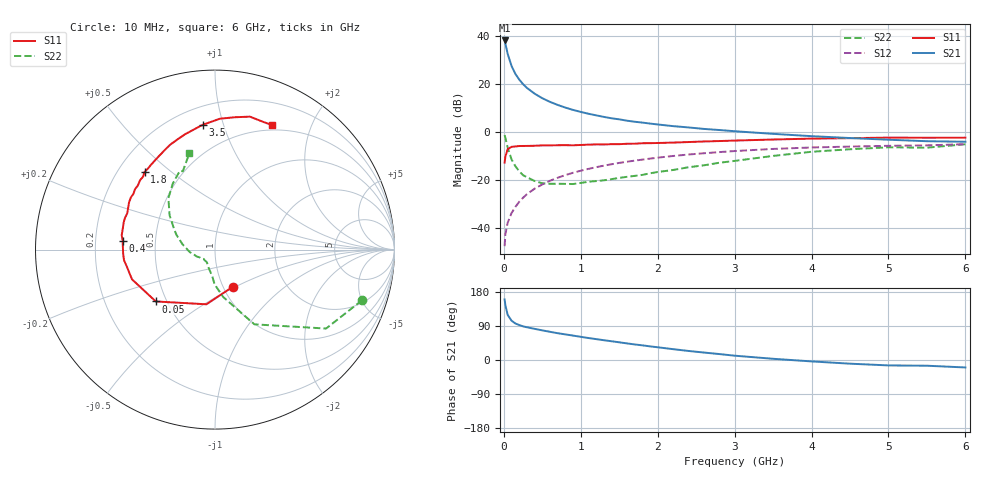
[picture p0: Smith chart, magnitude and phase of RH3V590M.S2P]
! SIEMENS Small Signal Semiconductors
! BFR106
! Si NPN RF Bipolar Junction Transistor in SOT23
! VCE = 3.5 V  IC = 90 mA
! Common Emitter S-Parameters:  August  1996
# GHz  S  MA  R  50
!  f  S11  S21  S12  S22
! GHz  MAG  ANG  MAG  ANG  MAG  ANG  MAG  ANG
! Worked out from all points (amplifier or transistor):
!   36 points, 10 MHz to 6 GHz, reference 50 ohm
!   highest |S21| = 38.3 dB at 10 MHz (marker M1)
!   |S21| within 3 dB of that: start of sweep to 31.7 MHz
!   unconditionally stable (mu >= 1): 167.4 MHz to 2.468 GHz; 5.445 GHz to end of sweep
!   at 250 MHz: K = 1.06, MAG = 22.3 dB, |S12| = -27.5 dB
!   at 1.4 GHz: K = 1.06, MAG = 8.1 dB, |S12| = -13.5 dB
!   at 6 GHz: K = 1.00, MAG = 0.3 dB, |S12| = -5.1 dB
!   S11 on the Smith chart (normalised r, x): 10 MHz: 1.11, -0.48; 50 MHz: 0.44, -0.31; 400 MHz: 0.32, +0.04; 1.8 GHz: 0.31, +0.41; 3.5 GHz: 0.31, +0.85; 6 GHz: 0.44, +1.47
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0.01  0.2292 -64.2  82.62 159.9  0.0041 78.1  0.8664 -19.0
0.02  0.3084 -98.9  70.99 144.5  0.0073 70.5  0.7594 -35.4
0.05  0.4385 -138.8  43.19 119.0  0.0127 63.4  0.4707 -62.2
0.1  0.4912 -160.3  24.21 103.7  0.0202 66.1  0.268 -80.2
0.15  0.5007 -169.3  16.5 96.4  0.0272 68.3  0.1932 -90.7
0.2  0.5104 -173.3  12.54 92.2  0.0348 71.5  0.1511 -95.6
0.25  0.5123 -177.4  10.06 88.8  0.0423 72.8  0.1252 -102.2
0.3  0.5129 179.5  8.403 86.4  0.0502 74.0  0.1137 -106.8
0.4  0.5171 174.5  6.368 82.2  0.0654 73.8  0.0947 -115.3
0.5  0.5261 171.2  5.108 78.2  0.0802 73.6  0.0849 -121.7
0.6  0.5268 167.3  4.283 74.4  0.0959 72.6  0.0828 -126.0
0.7  0.5307 163.5  3.699 70.7  0.1107 71.6  0.0829 -131.3
0.9  0.5292 157.5  2.908 64.4  0.141 68.8  0.0818 -140.5
1.1  0.5465 151.2  2.419 58.0  0.1698 66.0  0.0914 -147.1
1.4  0.5588 142.8  1.943 49.5  0.2122 61.3  0.1036 -157.0
1.8  0.5842 132.1  1.58 38.7  0.2655 55.1  0.1269 -170.0
2.2  0.6028 122.6  1.332 28.6  0.3161 48.6  0.1609 177.2
3  0.6638 104.6  1.042 11.4  0.4008 35.8  0.2494 154.6
3.5  0.6986 95.7  0.918 3.2  0.4441 28.1  0.3172 142.9
4.5  0.7461 81.3  0.75 -9.7  0.4971 13.5  0.437 122.5
5.5  0.7606 69.5  0.644 -15.1  0.5269 4.3  0.4719 112.3
6  0.7633 65.3  0.628 -19.7  0.5584 -2.6  0.5558 104.9
